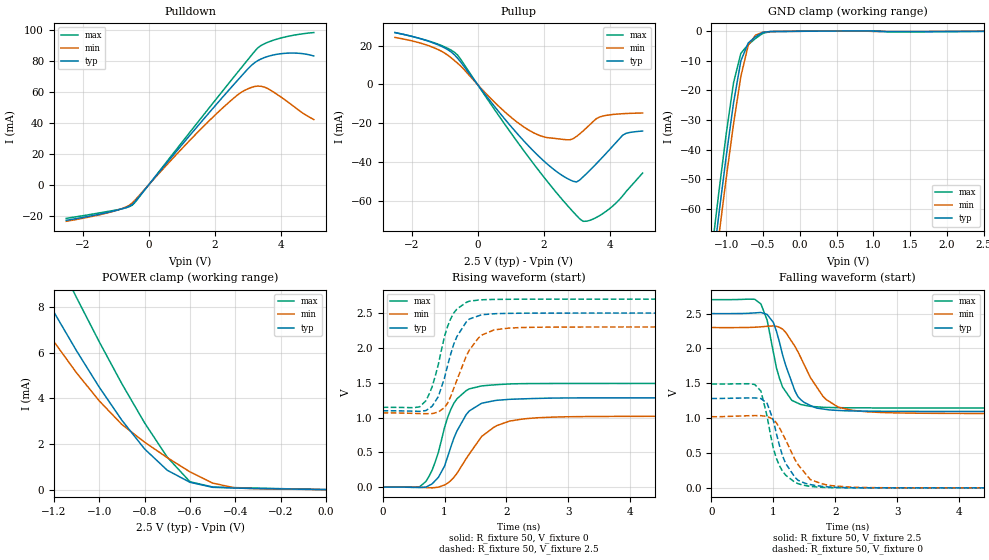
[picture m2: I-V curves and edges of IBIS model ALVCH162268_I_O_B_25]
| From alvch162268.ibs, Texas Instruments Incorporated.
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|************* ALVCH162268 OUTPUT (2.5 V) MODEL**************
[Model]   ALVCH162268_I_O_B_25
Model_type  I/O
Polarity   Non-Inverting
Enable   Active-Low
Vinl = 0.7V
Vinh = 1.7V
Vmeas = 1.25V
Cref = 30pF
Rref = 500
Vref = 0
| variable   typ   min   max
C_comp   8.15p   NA   NA
[Temperature Range]   50   100   0
[Voltage range]   2.5   2.3   2.7
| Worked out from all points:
|   slope of the pulldown table from 0 to 0.375 V, typ, clamps not added: 38.6 ohm
|   slope of the pullup table from 0 to 0.375 V, typ, clamps not added: 45.3 ohm
|   GND clamp passes 1 mA (typ) near -0.54 V on its own axis
|   POWER clamp passes 1 mA (typ) near -0.72 V on its own axis
|   rising waveform, R_fixture 50, V_fixture 0: 20-80 % time 368ps typ, 527ps min, 321ps max; typ from 0 V to 1.28 V
|   falling waveform, R_fixture 50, V_fixture 2.5: 20-80 % time 298ps typ, 472ps min, 242ps max; typ from 2.5 V to 1.1 V
|   rising waveform, R_fixture 50, V_fixture 2.5: 20-80 % time 312ps typ, 369ps min, 282ps max; typ from 1.1 V to 2.5 V
|   falling waveform, R_fixture 50, V_fixture 0: 20-80 % time 293ps typ, 392ps min, 258ps max; typ from 1.28 V to 0 V
|Process range|   weak   strong
[Pullup]
|   50C:2.5V:   100C:2.3V:weak   0C:2.7V:strong
|   Voltage   I(typ)   I(min)   I(max)
-2.5V     26.69mA    24.19mA    26.69mA
-1.3V     21.11mA    18.76mA    21.37mA
-600mV    13.45mA    10.88mA    15.07mA
800mV     -17.23mA   -13.66mA   -19.81mA
1.7V      -34.29mA   -24.83mA   -40.79mA
2.3V      -43.52mA   -27.64mA   -53.74mA
2.8V      -49.03mA   -28.43mA   -63.67mA
3V        -50.1mA    -26.67mA   -67.36mA
3.2V      -47.45mA   -23.85mA   -70.32mA
3.7V      -38.94mA   -16.69mA   -67.38mA
4.4V      -26.02mA   -15.01mA   -57.18mA
5V        -23.92mA   -14.65mA   -45.53mA
[Pulldown]
|   50C:2.5V:   100C:2.3V:weak   0C:2.7V:strong
|   Voltage   I(typ)   I(min)   I(max)
-2.5V     -22.93mA   -23.56mA   -21.65mA
-1.1V     -17.12mA   -17.3mA    -16.68mA
-700mV    -14.74mA   -14.42mA   -14.93mA
-500mV    -12.77mA   -11.76mA   -13.18mA
800mV     20.63mA    18.71mA    21.85mA
1.8V      45.82mA    40.72mA    48.86mA
2.6V      65.34mA    56.45mA    70.2mA
3V        74.79mA    61.96mA    80.76mA
3.3V      80.19mA    63.76mA    88.41mA
3.6V      82.9mA     62.24mA    92.03mA
4.3V      85.13mA    52.17mA    96.27mA
5V        83.23mA    42.16mA    98.35mA
[GND Clamp]
|   50C:2.5V:   100C:2.3V:weak   0C:2.7V:strong
|   Voltage   I(typ)   I(min)   I(max)
-2.5V     -364.6mA   -368.2mA   -360.4mA
-1.2V     -82.61mA   -89.67mA   -75.35mA
-1.1V     -62.17mA   -69.47mA   -54.65mA
-1V       -42.47mA   -49.89mA   -34.89mA
-900mV    -24.27mA   -31.4mA    -17.5mA
-800mV    -10.01mA   -15.26mA   -7.433mA
-700mV    -3.952mA   -4.72mA    -4.496mA
-600mV    -1.826mA   -1.304mA   -2.409mA
-500mV    -349.8uA   -297uA     -675.2uA
-400mV    -86.82uA   -82.46uA   -114.9uA
800mV     108.5uA    63.96uA    161.5uA
2.5V      123.5pA    21.94uA    -39.79uA
[POWER Clamp]
|   50C:2.5V:   100C:2.3V:weak   0C:2.7V:strong
|   Voltage   I(typ)   I(min)   I(max)
-2.5V     34.4mA     29.85mA    39.82mA
-1.4V     11.42mA    9.537mA    14.6mA
-1.3V     9.571mA    7.97mA     12.49mA
-1.2V     7.787mA    6.491mA    10.43mA
-1.1V     6.087mA    5.121mA    8.418mA
-900mV    3.039mA    2.854mA    4.637mA
-800mV    1.782mA    2.079mA    2.925mA
-700mV    847.1uA    1.4mA      1.42mA
-600mV    319.5uA    777.9uA    343.7uA
-500mV    100.8uA    285.5uA    113uA
-400mV    66.77uA    70.46uA    86.75uA
0V        121.4pA    549.5pA    66.34pA
[ramp]
| variable   typ   min   max
dV/dt_r   7.7288E-01/3.6991E-10  6.1853E-01/5.3015E-10  8.9577E-01/3.2164E-10
dV/dt_f   8.5121E-01/2.9758E-10  7.5397E-01/4.8061E-10  9.3662E-01/2.3805E-10
[Rising Waveform]
R_fixture = 50
V_fixture = 0
V_fixture_min = 0
V_fixture_max = 0
C_fixture = 0
L_fixture = 0
|   50C:2.5V:   100C:2.3V:weak   0C:2.7V:strong
|   Time   V(typ)   V(min)   V(max)
0s        0V         0V         0V
600ps     -5.867mV   -2.892mV   6.672mV
800ps     47.01mV    -10.32mV   243.7mV
1ns       301.3mV    30.93mV    856.1mV
1.15ns    701mV      138.1mV    1.203V
1.35ns    1.042V     408.7mV    1.386V
1.6ns     1.205V     727.5mV    1.454V
2.05ns    1.261V     948.3mV    1.482V
2.75ns    1.279V     1.005V     1.488V
13.5ns    1.282V     1.021V     1.489V
[Falling Waveform]
R_fixture = 50
V_fixture = 2.5
V_fixture_min = 2.3
V_fixture_max = 2.7
C_fixture = 0
L_fixture = 0
|   50C:2.5V:   100C:2.3V:weak   0C:2.7V:strong
|   Time   V(typ)   V(min)   V(max)
0s        2.5V       2.3V       2.7V
700ps     2.509V     2.304V     2.705V
900ps     2.487V     2.317V     2.406V
1ns       2.373V     2.323V     1.95V
1.15ns    1.907V     2.277V     1.446V
1.4ns     1.305V     1.949V     1.213V
1.6ns     1.182V     1.581V     1.169V
2.05ns    1.11V      1.157V     1.15V
2.7ns     1.099V     1.083V     1.147V
13.5ns    1.097V     1.066V     1.146V
[Rising Waveform]
R_fixture = 50
V_fixture = 2.5
V_fixture_min = 2.3
V_fixture_max = 2.7
C_fixture = 0
L_fixture = 0
|   50C:2.5V:   100C:2.3V:weak   0C:2.7V:strong
|   Time   V(typ)   V(min)   V(max)
0s        1.097V     1.066V     1.146V
600ps     1.089V     1.057V     1.154V
800ps     1.161V     1.056V     1.441V
900ps     1.3V       1.078V     1.762V
1.1ns     1.91V      1.303V     2.418V
1.2ns     2.162V     1.536V     2.558V
1.4ns     2.414V     1.967V     2.671V
1.6ns     2.476V     2.183V     2.691V
2.25ns    2.498V     2.292V     2.699V
13.5ns    2.5V       2.3V       2.7V
[Falling Waveform]
R_fixture = 50
V_fixture = 0
V_fixture_min = 0
V_fixture_max = 0
C_fixture = 0
L_fixture = 0
|   50C:2.5V:   100C:2.3V:weak   0C:2.7V:strong
|   Time   V(typ)   V(min)   V(max)
0s        1.282V     1.021V     1.489V
700ps     1.29V      1.037V     1.483V
800ps     1.281V     1.036V     1.388V
900ps     1.212V     1.023V     1.026V
1ns       969.8mV    982.9mV    567.4mV
1.1ns     606mV      861.1mV    316.9mV
1.35ns    151.1mV    405.6mV    79.22mV
1.6ns     46.55mV    116.7mV    20.29mV
2.75ns    452.6uV    1.97mV     168.1uV
13.5ns    3.281uV    654.1nV    2.772uV
